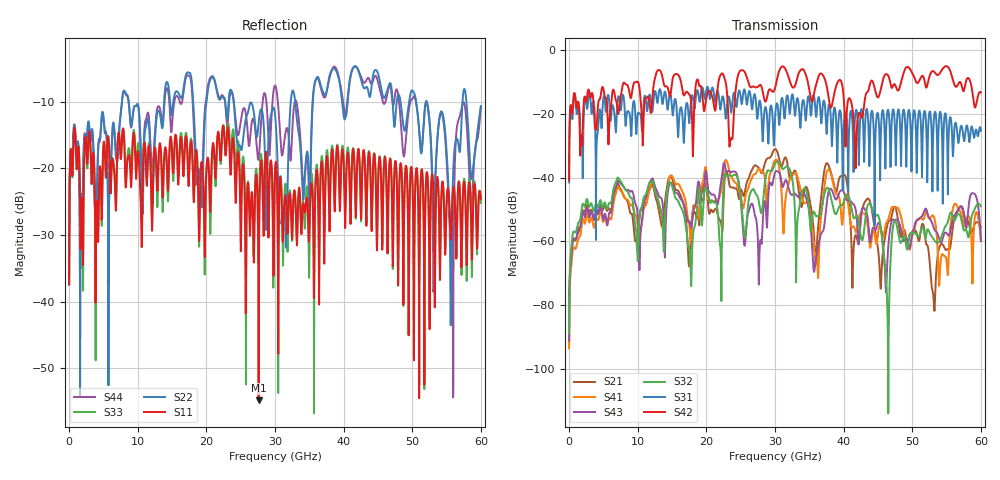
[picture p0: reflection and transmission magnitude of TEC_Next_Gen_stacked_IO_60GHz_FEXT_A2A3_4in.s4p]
!! CHANNEL DESCRIPTION:  Next Generation 28Gbps Press-fit Stacked I/O Connector
!!  with 4" 5-6-5 Megtron 6 Stripline trace on host side and 1.25" 7-5-7 Megtron 6 Microstrip trace on plug side
!! HOST PCB DESCRIPTION:  PCB thickness 3.425 mm
!!  26 Layer Board, 15 GND planes, 4 Layer route-out on Layers 7,11,17,21, 8mil stub on vias
!!  Pairs on following layers
!!  Layer 07 - A02A03 A14A15 D05D06
!!  Layer 11 - D020D3 C05C06 D14D15
!!  Layer 17 - C02C03 B05B06 C14C15
!!  Layer 21 - B02B03 A05A06 B14B15
!! CONNECTOR DESCRIPTION:  Next Generation 28Gbps Press-fit Stacked I/O Connector
!! PLUG-IN CARD DESCRIPTION:  PCB thickness 1mm thick
!!  6 Layer Board, 4 GND planes, 0.35 x 1.4mm mating pads
!!  Micro-strip diff traces referenced to GND plane 3mils down, 2nd GND plane 17mils from top of board
!!  PCB GND planes are symmetric
!! MODEL DESCRIPTION: TE Connectivity S-parameter model produced from Macro-model, Extracted .s4p FEXT (Victim B05B06 - Aggressor A02A03)
!! MODEL DATE: 5/15/2014 CR32f, FPR23
!! MODEL STATUS: Developmental
!! MODEL GEOMETRY: 4 Rows - Rows A, B, C, D. 3 pairs in each row, 12 total pairs
!! MODEL FREQUENCY RANGE: DC to 60 GHz in 10 MHz frequency steps
!! MODEL EDGE RATE LIMITATION: 8.33 ps (Using conservative 0.5/Fmax rule of thumb)
!! TIME-DOMAIN TRANSFORM CAUTIONS:
!! 1.) Do not simulate transient edge rates faster than the number listed above.  Edge
!!  rates faster than this number contain significant spectral content at frequencies
!!  above the model's highest frequency.
!! 2.) Even when simulating edge rates that are slower than the number listed above, be
!!  aware that the best time resolution possible with a direct iFFT is (1 / 2Fmax).
!!  As a result, time resolution is typically not adequate for most time-domain
!!  simulations unless tricks such as frequency-domain zero-padding and windowing are
!!  used to minimize leakage and aliasing.
!! 3.) Because the model has a uniform frequency step, a direct iFFT will result in an
!!  impulse that that has a time length given by either (1 / Fstep) or (1 / 2Fstep),
!!  depending on the transform being used.  Care has been taken in selecting the
!!  frequency step to ensure a settled impulse response for the model.  Therefore,
!!  convolution with the model's impulse response should present no issues.  However,
!!  if directly concatenating s-parameter models in the frequency domain a user must
!!  either interpolate necessary interim frequencies or complete impulse response
!!  zero-padding.  Impulse response zero-padding is more difficult, but more accurate.
!! PORT DEFINITIONS:
!! Port  1  ----->  Host A02		B05 Module <-----  Port  2
!! Port  3  ----->  Host A03		B06 Module <-----  Port  4
! Touchstone data
! Created: 29-Sep-2014 by IdEM R2011 (7.0.3)
# Hz S MA R 50
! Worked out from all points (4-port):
!   6000 points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, 10 MHz to 60 GHz, reference 50 ohm
!   strongest paths, dB at 10 MHz, 15.01 GHz, 30.01 GHz, 45.01 GHz, 60 GHz:
!     S42: -41.0, -10.1, -12.0, -14.9, -13.4
!     S31: -41.5, -18.4, -21.3, -20.0, -25.4
!     S32: -88.9, -42.6, -35.7, -51.8, -49.0
!     S43: -91.1, -41.9, -38.3, -54.4, -59.9
!     S41: -93.5, -39.6, -34.6, -57.5, -59.8
!     S21: -91.0, -40.2, -31.1, -62.2, -55.6
!   lowest |S11| = -54.8 dB at 27.62 GHz (marker M1), VSWR 1.00, Z = 49.9 - j0.107 ohm
!   |S11| at or under -10 dB: start of sweep to end of sweep
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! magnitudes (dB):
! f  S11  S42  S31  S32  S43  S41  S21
! 10 MHz  -37.4  -41.0  -41.5  -88.9  -91.1  -93.5  -91.0
! 7.24 GHz  -14.6  -19.4  -14.5  -40.2  -41.1  -43.1  -42.4
! 17.47 GHz  -21.8  -13.9  -22.5  -62.0  -53.8  -54.0  -67.7
! 27.62 GHz  -54.8  -11.3  -17.4  -47.2  -70.9  -37.2  -36.9
! 43.82 GHz  -18.6  -10.9  -28.8  -48.2  -59.9  -61.6  -47.4
! 46.44 GHz  -30.7  -7.9  -18.8  -87.5  -63.8  -53.4  -54.3
! 60 GHz  -24.6  -13.4  -25.4  -49.0  -59.9  -59.8  -55.6
